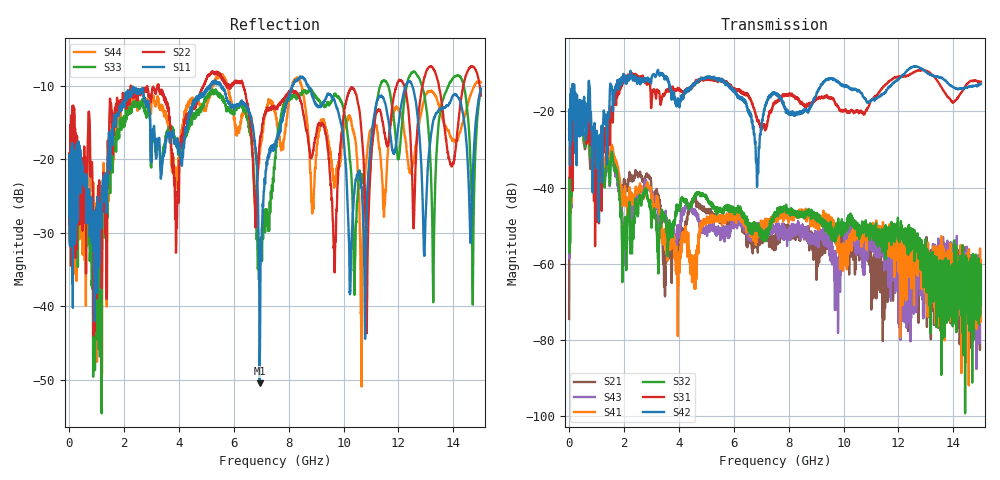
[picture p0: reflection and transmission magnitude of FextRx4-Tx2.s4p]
! FILE: N:\QM 2007\Prüfprotokolle\Highspeed\Konfektionierte Ltg\L45593-D106\D30\8216\0002\Fext\FextRx4-Tx2.s4p
# MHz S DB R 50.00
! FREQ  S11  S12  S13  S14
!  S21  S22  S23  S24
!  S31  S32  S33  S34
!  S41  S42  S43  S44
!  DB  ANG  DB  ANG  DB  ANG  DB  ANG
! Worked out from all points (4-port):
!   2999 points, 10 MHz to 15 GHz, reference 50 ohm
!   strongest paths, dB at 10 MHz, 3.755 GHz, 7.505 GHz, 11.26 GHz, 15 GHz:
!     S42: -24.7, -15.4, -15.2, -16.2, -12.9
!     S31: -24.5, -13.8, -17.8, -15.4, -12.2
!     S32: -46.8, -50.5, -47.7, -51.1, -70.6
!     S41: -53.1, -53.1, -48.9, -53.5, -59.2
!     S43: -49.6, -50.9, -50.7, -55.6, -61.0
!     S21: -74.5, -59.4, -53.3, -54.6, -66.0
!   lowest |S11| = -50.4 dB at 6.945 GHz (marker M1), VSWR 1.01, Z = 49.9 - j0.279 ohm
!   |S11| at or under -10 dB: start of sweep to 5.122 GHz; 5.537 GHz to 8.129 GHz (2.592 GHz wide, 37.9 % of centre); 8.716 GHz to 12.26 GHz (3.549 GHz wide, 33.8 % of centre)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
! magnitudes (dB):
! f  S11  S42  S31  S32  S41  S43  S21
! 10 MHz  -19.4  -24.7  -24.5  -46.8  -53.1  -49.6  -74.5
! 360 MHz  -24.3  -19.8  -22.7  -23.6  -23.8  -24.2  -23.9
! 3.98 GHz  -19.0  -16.8  -14.2  -45.1  -65.6  -52.1  -53.9
! 6.945 GHz  -50.4  -27.9  -23.1  -51.1  -50.7  -49.8  -53.5
! 8.28 GHz  -9.3  -20.4  -16.7  -46.5  -47.2  -50.5  -51.8
! 10.65 GHz  -23.8  -15.3  -19.9  -51.1  -52.9  -56.7  -56.3
! 15 GHz  -10.4  -12.9  -12.2  -70.6  -59.2  -61.0  -66.0
